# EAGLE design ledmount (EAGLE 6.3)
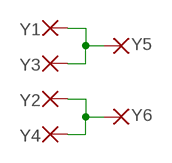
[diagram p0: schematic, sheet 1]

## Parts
Y1  SMD5  [SMD2,54-5,08]
Y2  SMD5  [SMD2,54-5,08]
Y3  SMD5  [SMD2,54-5,08]
Y4  SMD5  [SMD2,54-5,08]
Y5  SMD5  [SMD2,54-5,08]
Y6  SMD5  [SMD2,54-5,08]

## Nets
N$1: Y2.1(P) Y4.1(P) Y6.1(P)
N$2: Y1.1(P) Y3.1(P) Y5.1(P)

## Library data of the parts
Y1-Y6 = wirepad:SMD5: SMD PAD

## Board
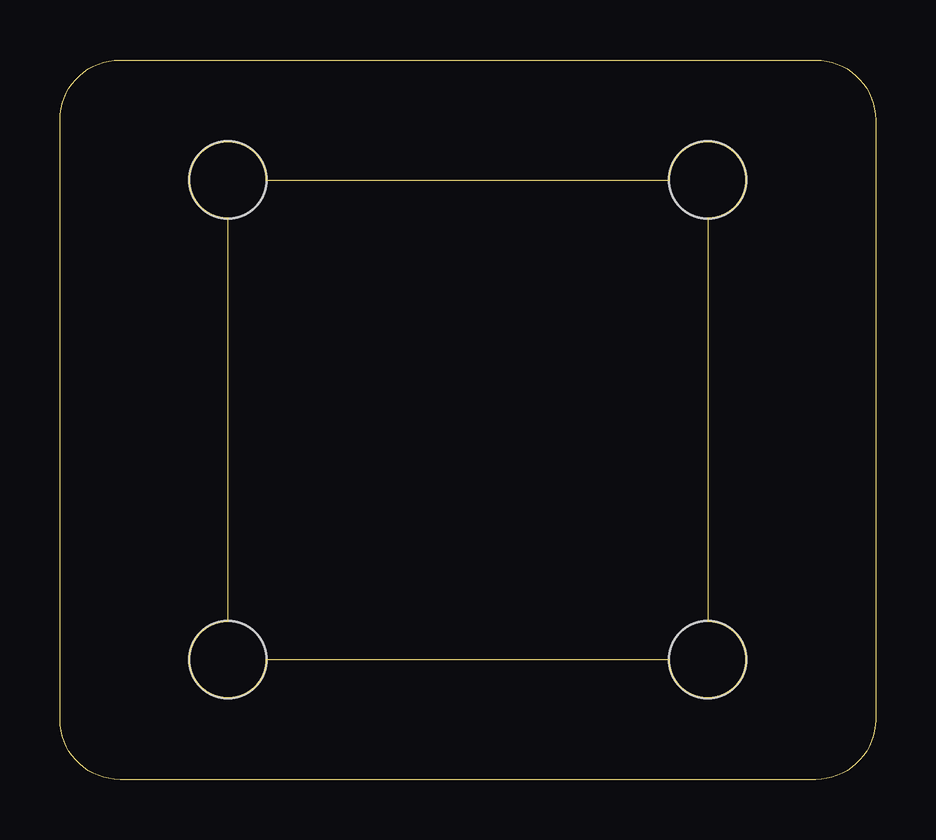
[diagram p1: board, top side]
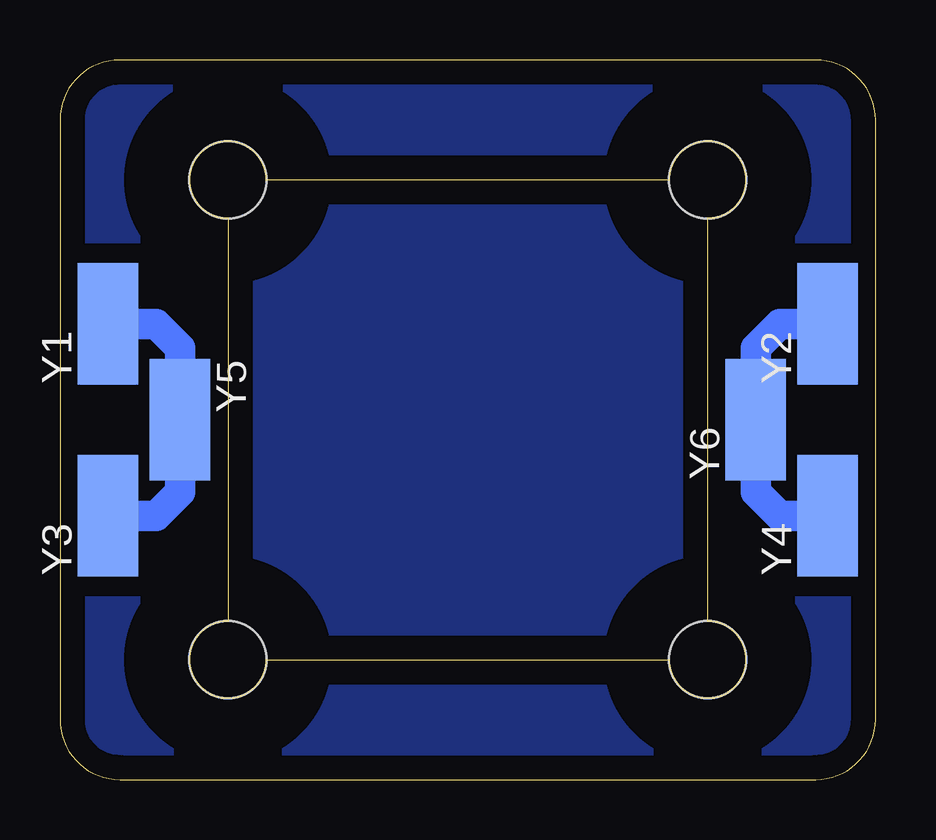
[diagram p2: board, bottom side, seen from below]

Size 34 x 30 mm. Coordinates in mm from the lower left corner, seen from the top.
Outline: 7,6.6 7,23.4 arc-270 8.6,25 25.4,25 arc-270 27,23.4 27,6.6 arc-270 25.4,5 8.6,5 arc-270 7,6.6
Outline: 0,2.5 0,27.5 arc-90 2.5,30 31.5,30 arc-90 34,27.5 34,2.5 arc-90 31.5,0 2.5,0 arc-90 0,2.5
Copper layers (1*16): Top 0.035mm / dielectric 1.5mm / Bottom 0.035mm
Design rules "default": minimum track width 10mil, minimum drill 24mil, track to track 8mil, track to pad 8mil, pad to pad 8mil, via to via 8mil, smd to smd 8mil, copper to edge 40mil, drill to drill 8mil, minimum pad ring 10mil, minimum via ring 8mil, stop-mask expansion 4mil, vias tented up to drill 0mil, thermal gap 10mil
Holes 3.2 mm at 7,25 27,25 27,5 7,5
bRestrict: area 3.5,21.5 to 10.5,28.5; area 23.5,21.5 to 30.5,28.5; area 23.5,1.5 to 30.5,8.5; area 3.5,1.5 to 10.5,8.5

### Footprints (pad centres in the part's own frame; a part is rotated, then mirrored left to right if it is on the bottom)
SMD2,54-5,08 = smd 2.54 x 5.08: 1 0,0

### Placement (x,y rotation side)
Y1  32,19 0 bottom
Y2  2,19 0 bottom
Y3  32,11 0 bottom
Y4  2,11 0 bottom
Y5  29,15 180 bottom
Y6  5,15 0 bottom

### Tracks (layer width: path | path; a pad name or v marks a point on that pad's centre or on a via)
N$1
  Bottom 1.27: Y2.1 4,19 5,18 Y6.1 5,12 4,11 Y4.1
N$2
  Bottom 1.27: Y1.1 30,19 29,18 Y5.1 29,12 30,11 Y3.1
N$3
  pour Bottom (isolate 0.813): 0,30 34,30 34,22 27,22 27,8 34,8 34,0 0,0 0,8 7,8 7,22 0,22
